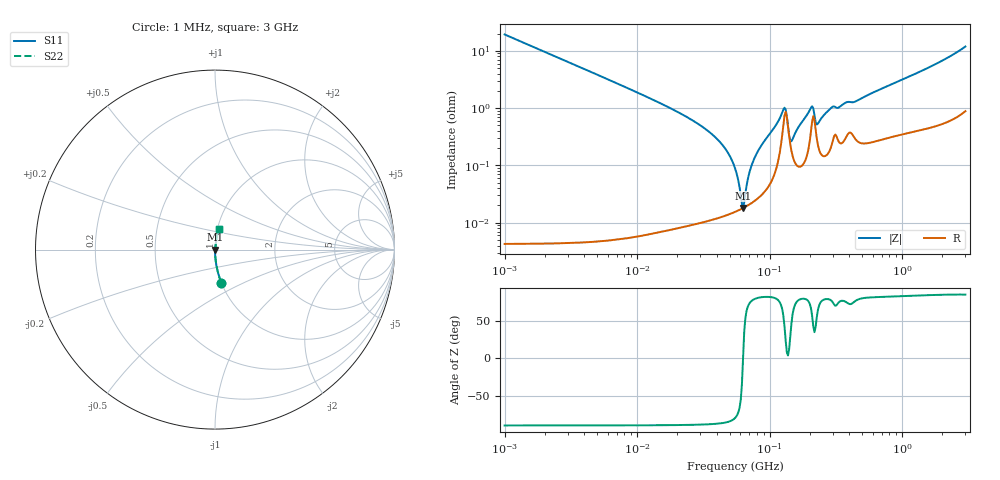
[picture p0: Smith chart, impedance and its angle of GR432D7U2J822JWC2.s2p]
!Murata Part Number: GR432D7U2J822JWC2
!These Parameters are Measured in Series Mode Connection
!Data Generated on Jun 10, 2025
!  o--ll--o
!Port1  Port2
!  o------o
!Operation Temp=25[degC], DC Bias Voltage=0[V]
!Freq. Start=1000[kHz] Stop=3[GHz] 401[Steps]
# Hz S RI R 50
!Freq.(Hz) S11(Real) S11(Imag) S21(Real) S21(Imag) S12(Real) S12(Imag) S22(Real) S22(Imag)
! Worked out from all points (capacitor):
!   401 points, 1 MHz to 3 GHz, reference 50 ohm
!   read as one part in series: C = 8.25 nF near 1.041 MHz
!   lowest |Z| = 18 mohm at 63.01 MHz (marker M1)
!   series resonance near 62.97 MHz, so ESL is about 770 pH
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1000000  0.0359 -0.1859  0.9641 0.1859  0.9641 0.1859  0.0359 -0.1859
3823119  0.00256 -0.0501  0.9974 0.0501  0.9974 0.0501  0.00256 -0.0501
1.461624e7  0.000224 -0.0125  0.9998 0.0125  0.9998 0.0125  0.000224 -0.0125
3.670325e7  0.000124 -0.0035  0.9999 0.0035  0.9999 0.0035  0.000124 -0.0035
4.666789e7  0.000137 -0.0019  0.9999 0.0019  0.9999 0.0019  0.000137 -0.0019
5.477226e7  0.000155 -0.000882  0.9998 0.000882  0.9998 0.000882  0.000155 -0.000882
6.053752e7  0.000172 -0.00025  0.9998 0.00025  0.9998 0.00025  0.000172 -0.00025
6.301011e7  0.00018 4.6e-06  0.9998 -4.6e-06  0.9998 -4.6e-06  0.00018 4.6e-06
6.558369e7  0.000189 0.000262  0.9998 -0.000262  0.9998 -0.000262  0.000189 0.000262
7.105049e7  0.000212 0.000787  0.9998 -0.000787  0.9998 -0.000787  0.000212 0.000787
7.697298e7  0.000242 0.00133  0.9998 -0.00133  0.9998 -0.00133  0.000242 0.00133
1.269575e8  0.00517 0.00785  0.9948 -0.00785  0.9948 -0.00785  0.00517 0.00785
1.321429e8  0.00858 0.00373  0.9914 -0.00373  0.9914 -0.00373  0.00858 0.00373
1.403209e8  0.00324 0.000701  0.9968 -0.000701  0.9968 -0.000701  0.00324 0.000701
1.460522e8  0.0018 0.00193  0.9982 -0.00193  0.9982 -0.00193  0.0018 0.00193
2.011837e8  0.00282 0.00887  0.9972 -0.00887  0.9972 -0.00887  0.00282 0.00887
2.094008e8  0.00595 0.00889  0.994 -0.00889  0.994 -0.00889  0.00595 0.00889
2.314421e8  0.00227 0.00487  0.9977 -0.00487  0.9977 -0.00487  0.00227 0.00487
2.942768e8  0.00239 0.00999  0.9976 -0.00999  0.9976 -0.00999  0.00239 0.00999
4.391493e8  0.00313 0.0125  0.9969 -0.0125  0.9969 -0.0125  0.00313 0.0125
8.005644e8  0.00366 0.0247  0.9963 -0.0247  0.9963 -0.0247  0.00366 0.0247
3e9  0.0222 0.1147  0.9778 -0.1147  0.9778 -0.1147  0.0222 0.1147
